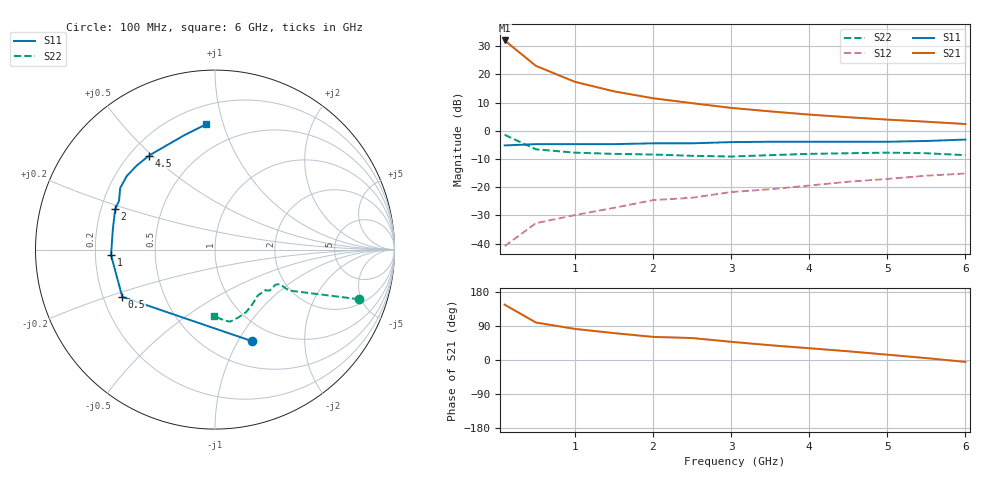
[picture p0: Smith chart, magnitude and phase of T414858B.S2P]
!AT-41485
!S-PARAMETERS at Vce=8V  Ic=25mA.  LAST UPDATED 07-21-92
# ghz s ma r 50
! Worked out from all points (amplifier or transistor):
!   13 points, 100 MHz to 6 GHz, reference 50 ohm
!   highest |S21| = 32.0 dB at 100 MHz (marker M1)
!   |S21| within 3 dB of that: start of sweep to 233.4 MHz
!   unconditionally stable (mu >= 1): 930.6 MHz to 5.004 GHz
!   at 1 GHz: K = 1.05, MAG = 22.3 dB, |S12| = -29.9 dB
!   at 3 GHz: K = 1.16, MAG = 12.5 dB, |S12| = -21.7 dB
!   at 6 GHz: K = 0.87, MSG = 8.8 dB, |S12| = -15.1 dB
!   S11 on the Smith chart (normalised r, x): 100 MHz: 0.78, -1.15; 500 MHz: 0.28, -0.22; 1 GHz: 0.27, -0.02; 2 GHz: 0.26, +0.18; 4.5 GHz: 0.28, +0.49; 6 GHz: 0.32, +0.88
0.1  0.55 -68.0  40.01 146.0  0.009 57.0  0.85 -19.0
0.5  0.58 -153.0  14.2 99.0  0.023 52.0  0.47 -29.0
1  0.58 -177.0  7.39 82.0  0.032 63.0  0.41 -28.0
1.5  0.58 169.0  5.01 71.0  0.043 60.0  0.39 -30.0
2  0.6 158.0  3.78 61.0  0.059 64.0  0.38 -37.0
2.5  0.6 153.0  3.09 58.0  0.065 71.0  0.36 -39.0
3  0.63 147.0  2.55 48.0  0.082 68.0  0.35 -47.0
3.5  0.64 140.0  2.21 39.0  0.092 67.0  0.37 -56.0
4  0.64 133.0  1.94 31.0  0.107 65.0  0.39 -64.0
4.5  0.64 125.0  1.74 23.0  0.125 63.0  0.4 -71.0
5  0.64 115.0  1.58 14.0  0.14 56.0  0.41 -78.0
5.5  0.66 105.0  1.45 5.0  0.16 50.0  0.4 -82.0
6  0.7 94.0  1.32 -5.0  0.175 47.0  0.37 -91.0
